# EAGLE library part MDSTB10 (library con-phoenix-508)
PHOENIX
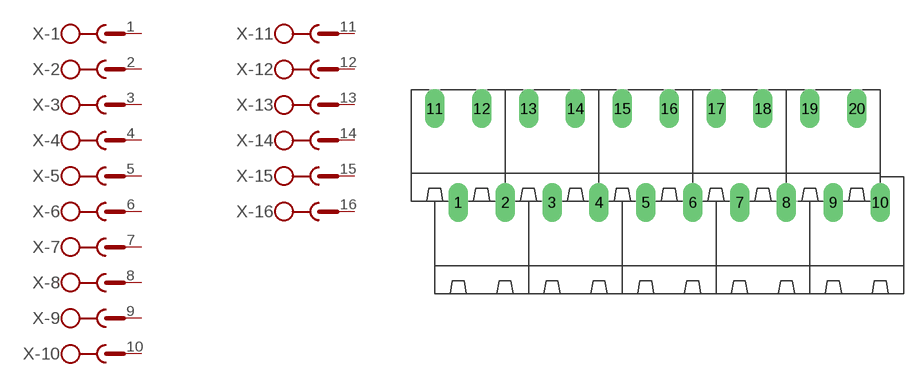
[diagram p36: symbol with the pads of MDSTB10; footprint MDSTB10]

Designator prefix X; gates -1=SK -2=SK -3=SK -4=SK -5=SK -6=SK -7=SK -8=SK -9=SK -10=SK -11=SK -12=SK -13=SK -14=SK -15=SK -16=SK -17=SK -18=SK -19=SK -20=SKV

## MDSTB10 (OC_FARNELL: unknown; OC_NEWARK: unknown)  [MDSTB10]
1  -1:1  pas
2  -2:1  pas
3  -3:1  pas
4  -4:1  pas
5  -5:1  pas
6  -6:1  pas
7  -7:1  pas
8  -8:1  pas
9  -9:1  pas
10  -10:1  pas
11  -11:1  pas
12  -12:1  pas
13  -13:1  pas
14  -14:1  pas
15  -15:1  pas
16  -16:1  pas
17  -17:1  pas
18  -18:1  pas
19  -19:1  pas
20  -20:1  pas

## Footprint MDSTB10 (pad centres in mm)
PHOENIX
drill 1.397 long: 1 -21.59,-5.08; 2 -16.51,-5.08; 3 -11.43,-5.08; 4 -6.35,-5.08; 5 -1.27,-5.08; 6 3.81,-5.08; 7 8.89,-5.08; 8 13.97,-5.08; 9 19.05,-5.08; 10 24.13,-5.08; 11 -24.13,5.08; 12 -19.05,5.08; 13 -13.97,5.08; 14 -8.89,5.08; 15 -3.81,5.08; 16 1.27,5.08; 17 6.35,5.08; 18 11.43,5.08; 19 16.51,5.08; 20 21.59,5.08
